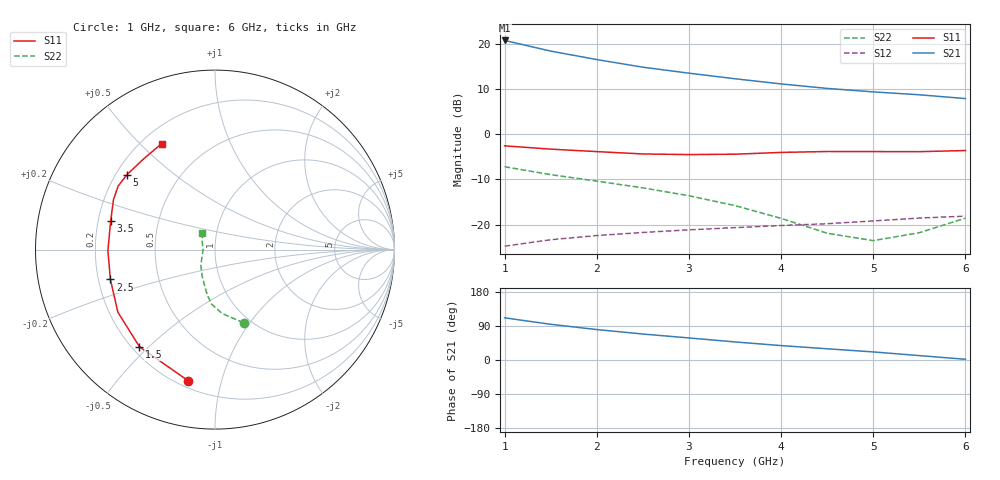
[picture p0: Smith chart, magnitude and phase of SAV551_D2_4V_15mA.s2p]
! Created Mon Oct 27 14:30:53 2008
# hz S ma R 50
! 2 Port Network Data from SP1.SP block
! freq  magS11  angS11  magS21  angS21  magS12  angS12  magS22  angS22
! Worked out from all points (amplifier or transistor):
!   11 points, 1 GHz to 6 GHz, reference 50 ohm
!   highest |S21| = 20.8 dB at 1 GHz (marker M1)
!   |S21| within 3 dB of that: start of sweep to 1.672 GHz
!   unconditionally stable (mu >= 1): 4.439 GHz to end of sweep
!   at 1.5 GHz: K = 0.46, MSG = 20.9 dB, |S12| = -23.4 dB
!   at 3.5 GHz: K = 0.91, MSG = 16.5 dB, |S12| = -20.7 dB
!   at 6 GHz: K = 1.08, MAG = 11.3 dB, |S12| = -18.1 dB
!   S11 on the Smith chart (normalised r, x): 1 GHz: 0.24, -0.79; 1.5 GHz: 0.23, -0.47; 2.5 GHz: 0.25, -0.13; 3.5 GHz: 0.25, +0.12; 5 GHz: 0.24, +0.35; 6 GHz: 0.28, +0.58
1e9  0.7453 -101.6  10.97 111.3  0.05768 39.5  0.4375 -68.7
1.5e9  0.6856 -127.9  8.362 94.2  0.06798 31.4  0.3578 -83.8
2e9  0.6437 -147.2  6.737 80.3  0.07556 25.4  0.3032 -93.8
2.5e9  0.6062 -164.1  5.544 68.5  0.08187 21.5  0.2553 -99.8
3e9  0.5967 -179.5  4.76 58.2  0.0875 17.9  0.2089 -106.1
3.5e9  0.6024 164.9  4.128 47.7  0.09251 14.0  0.1624 -116.4
4e9  0.6305 153.8  3.619 38.0  0.09771 10.8  0.1172 -132.3
4.5e9  0.6454 146.7  3.227 29.6  0.1023 8.5  0.08025 -153.3
5e9  0.644 139.6  2.953 21.3  0.1098 5.9  0.06642 -179.6
5.5e9  0.6429 128.7  2.743 11.6  0.1181 1.7  0.08129 150.5
6e9  0.6614 116.7  2.491 1.9  0.1241 -3.0  0.1179 127.6
